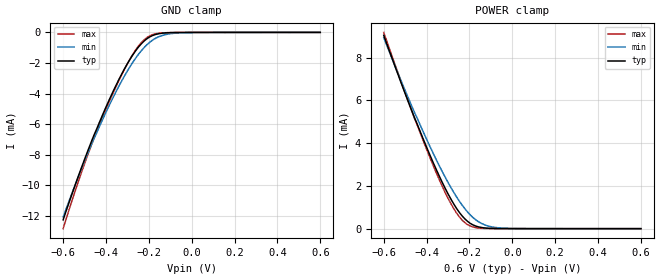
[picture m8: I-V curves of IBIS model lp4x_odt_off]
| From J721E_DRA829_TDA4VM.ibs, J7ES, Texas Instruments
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|   Model lp4x_odt_off
[Model] lp4x_odt_off
Model_type Input
Polarity   Non-Inverting
Enable   Active-High
Vinl =  0.0V
Vinh =  0.900V
C_comp   3.172pF   2.936pF   3.402pF
[Model Spec]
Vinh   0.900V   0.900V   0.900V
Vinl   0.0V   0.0V   0.0V
[Temperature Range]   25.000   0.125k   -40.000
[Voltage Range]   0.600V   0.570V   0.650V
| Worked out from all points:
|   GND clamp passes 1 mA (typ) near -0.25 V on its own axis
|   POWER clamp passes 1 mA (typ) near -0.26 V on its own axis
[GND_clamp]
|Voltage   I(typ)   I(min)   I(max)
-600mV    -12.26mA   -12.07mA   -12.83mA
-535mV    -9.631mA   -9.657mA   -9.999mA
-483mV    -7.674mA   -7.84mA    -7.926mA
-457mV    -6.749mA   -6.974mA   -6.957mA
-378mV    -4.198mA   -4.571mA   -4.306mA
-326mV    -2.706mA   -3.156mA   -2.747mA
-287mV    -1.735mA   -2.22mA    -1.722mA
-248mV    -949.8uA   -1.424mA   -887.8uA
-209mV    -414uA     -806.5uA   -336.6uA
-157mV    -95.46uA   -302uA     -61.63uA
-78.26mV  -9.093uA   -53uA      -8.171uA
600mV     0A         0A         0A
[POWER_clamp]
|Voltage   I(typ)   I(min)   I(max)
-600mV    9.037mA    8.928mA    9.175mA
-457mV    5.197mA    5.441mA    5.166mA
-352mV    2.698mA    3.164mA    2.544mA
-313mV    1.878mA    2.4mA      1.683mA
-274mV    1.164mA    1.707mA    946.8uA
-248mV    770.5uA    1.297mA    560.4uA
-222mV    461.8uA    938.4uA    283.8uA
-196mV    246uA      638.8uA    120.5uA
-157mV    79.32uA    316.3uA    23.54uA
-117mV    22.66uA    136.3uA    6.084uA
-78.26mV  6.704uA    54.45uA    1.893uA
600mV     0A         0A         0A
